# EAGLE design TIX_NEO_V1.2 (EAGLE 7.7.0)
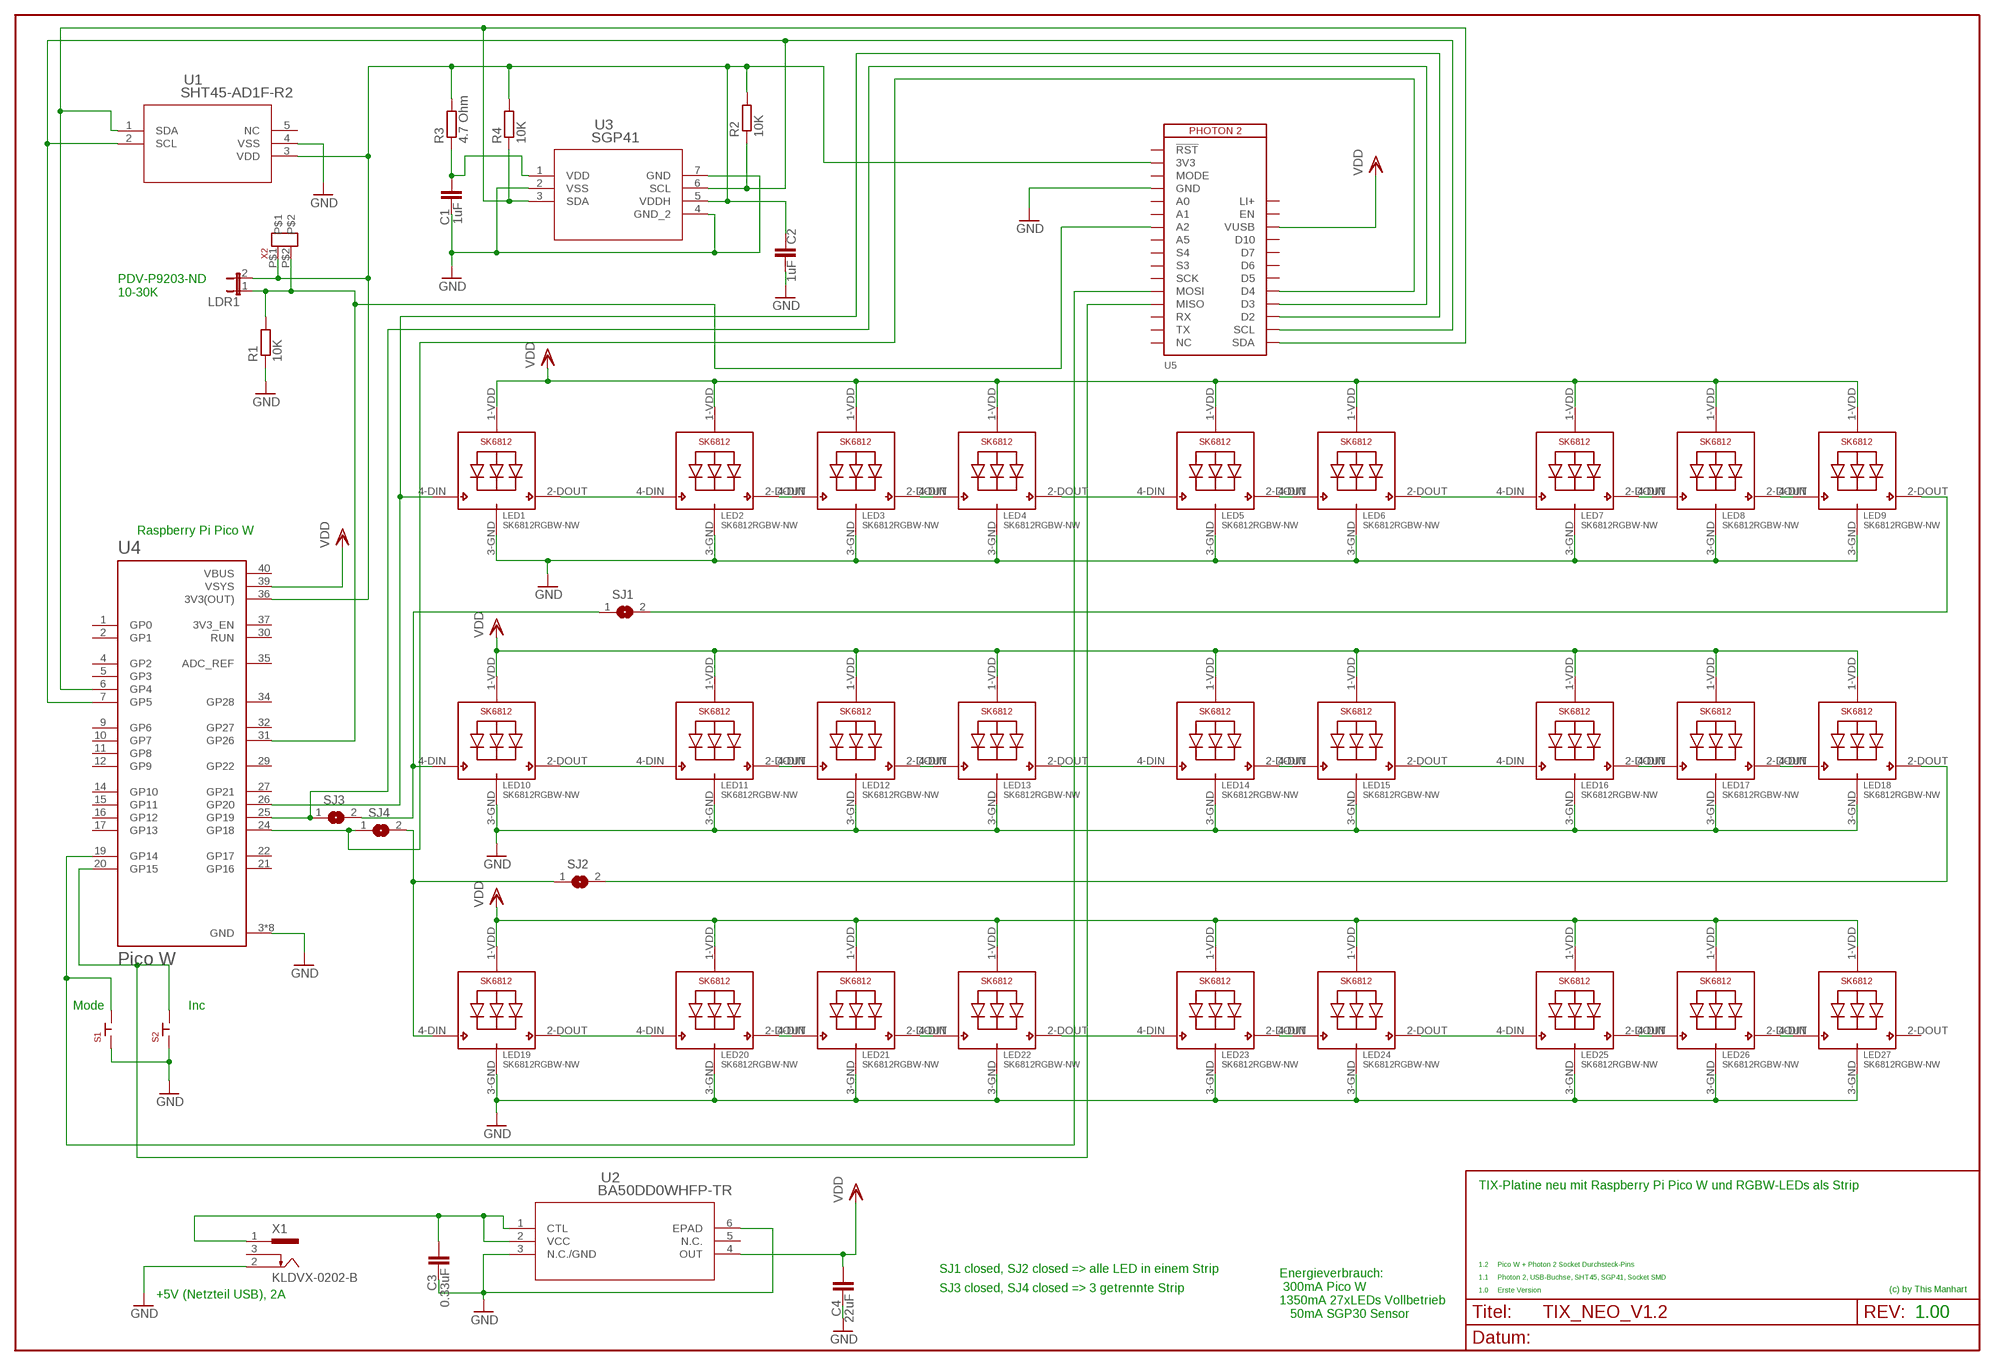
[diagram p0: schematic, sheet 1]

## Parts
C1  1uF  C-EUC0805  [C0805]
C2  1uF  C-EUC0805  [C0805]
C3  0.33uF  C-EUC0805  [C0805]
C4  22uF  C-EUC0805  [C0805]
LDR1  JUMPER_2P  [JUMPER_2P_2.54]
LED1  SK6812RGBW-NW  SK6812_5050W  [LED5050_W]
LED2  SK6812RGBW-NW  SK6812_5050W  [LED5050_W]
LED3  SK6812RGBW-NW  SK6812_5050W  [LED5050_W]
LED4  SK6812RGBW-NW  SK6812_5050W  [LED5050_W]
LED5  SK6812RGBW-NW  SK6812_5050W  [LED5050_W]
LED6  SK6812RGBW-NW  SK6812_5050W  [LED5050_W]
LED7  SK6812RGBW-NW  SK6812_5050W  [LED5050_W]
LED8  SK6812RGBW-NW  SK6812_5050W  [LED5050_W]
LED9  SK6812RGBW-NW  SK6812_5050W  [LED5050_W]
LED10  SK6812RGBW-NW  SK6812_5050W  [LED5050_W]
LED11  SK6812RGBW-NW  SK6812_5050W  [LED5050_W]
LED12  SK6812RGBW-NW  SK6812_5050W  [LED5050_W]
LED13  SK6812RGBW-NW  SK6812_5050W  [LED5050_W]
LED14  SK6812RGBW-NW  SK6812_5050W  [LED5050_W]
LED15  SK6812RGBW-NW  SK6812_5050W  [LED5050_W]
LED16  SK6812RGBW-NW  SK6812_5050W  [LED5050_W]
LED17  SK6812RGBW-NW  SK6812_5050W  [LED5050_W]
LED18  SK6812RGBW-NW  SK6812_5050W  [LED5050_W]
LED19  SK6812RGBW-NW  SK6812_5050W  [LED5050_W]
LED20  SK6812RGBW-NW  SK6812_5050W  [LED5050_W]
LED21  SK6812RGBW-NW  SK6812_5050W  [LED5050_W]
LED22  SK6812RGBW-NW  SK6812_5050W  [LED5050_W]
LED23  SK6812RGBW-NW  SK6812_5050W  [LED5050_W]
LED24  SK6812RGBW-NW  SK6812_5050W  [LED5050_W]
LED25  SK6812RGBW-NW  SK6812_5050W  [LED5050_W]
LED26  SK6812RGBW-NW  SK6812_5050W  [LED5050_W]
LED27  SK6812RGBW-NW  SK6812_5050W  [LED5050_W]
R1  10K  R-EU_R0805  [R0805]
R2  10K  R-EU_R0805  [R0805]
R3  4.7 Ohm  R-EU_R0805  [R0805]
R4  10K  R-EU_R0805  [R0805]
S1  TS02-66-170-BK-100-SCR-D  SCHURTER_LSH_PUSH_KEYDIP  [SCHURTER_LPH_PUSH_KEY]
S2  TS02-66-170-BK-100-SCR-D  SCHURTER_LSH_PUSH_KEYDIP  [SCHURTER_LPH_PUSH_KEY]
SJ1  SJ  [SJ]
SJ2  SJ  [SJ]
SJ3  SJ  [SJ]
SJ4  SJ  [SJ]
U1  SHT45-AD1F-R2  SHT40-AD1B-R2SHT4X_SEN-M  [SHT4X_SEN-M]
U2  BA50DD0WHFP-TR  BA50DD0WHFP-TRHRP5_ROM-M  [HRP5_ROM-M]
U3  SGP41  SGP41-D-R4DFN_SGP41-D-R4_SEN-M  [DFN_SGP41-D-R4_SEN-M]
U4  Pico W  RASPBERRY_PICO-NO_DEBUGW  [PICO-W]
U5  PHOTON2MM  [PHOTON2-MM]
X1  KLDVX-0202-B  [KLDVX-0202-B]
X2  PHOENIX_MPT_KLEMME_2P  [PHOENIX_MPT_KLEMME]

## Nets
GND: C1.1 C2.1 C3.1 C4.1 LED1.3-GND(GND) LED2.3-GND(GND) LED3.3-GND(GND) LED4.3-GND(GND) LED5.3-GND(GND) LED6.3-GND(GND) LED7.3-GND(GND) LED8.3-GND(GND) LED9.3-GND(GND) LED10.3-GND(GND) LED11.3-GND(GND) LED12.3-GND(GND) LED13.3-GND(GND) LED14.3-GND(GND) LED15.3-GND(GND) LED16.3-GND(GND) LED17.3-GND(GND) LED18.3-GND(GND) LED19.3-GND(GND) LED20.3-GND(GND) LED21.3-GND(GND) LED22.3-GND(GND) LED23.3-GND(GND) LED24.3-GND(GND) LED25.3-GND(GND) LED26.3-GND(GND) LED27.3-GND(GND) R1.1 S1.P$1 S2.P$1 U1.4(VSS) U2.3(N.C./GND) U2.6(EPAD) U3.2(VSS) U3.4(GND_2) U3.7(GND) U4.3(GND) U4.8(GND) U4.13(GND) U4.18(GND) U4.23(GND) U4.28(GND) U4.33(GND) U4.38(GND) U5.4(GND) X1.2
N$1: LED1.2-DOUT(DO) LED2.4-DIN(DI)
N$2: LED20.2-DOUT(DO) LED21.4-DIN(DI)
N$3: LED1.4-DIN(DI) U4.26(GP20) U5.19(D2)
N$4: LED2.2-DOUT(DO) LED3.4-DIN(DI)
N$5: LED3.2-DOUT(DO) LED4.4-DIN(DI)
N$6: LED4.2-DOUT(DO) LED5.4-DIN(DI)
N$7: LED5.2-DOUT(DO) LED6.4-DIN(DI)
N$8: LED6.2-DOUT(DO) LED7.4-DIN(DI)
N$9: LED7.2-DOUT(DO) LED8.4-DIN(DI)
N$10: LED8.2-DOUT(DO) LED9.4-DIN(DI)
N$11: LED9.2-DOUT(DO) SJ1.2
N$12: LED10.2-DOUT(DO) LED11.4-DIN(DI)
N$13: LED21.2-DOUT(DO) LED22.4-DIN(DI)
N$14: LED22.2-DOUT(DO) LED23.4-DIN(DI)
N$15: LED11.2-DOUT(DO) LED12.4-DIN(DI)
N$16: LED12.2-DOUT(DO) LED13.4-DIN(DI)
N$17: LED13.2-DOUT(DO) LED14.4-DIN(DI)
N$18: LED14.2-DOUT(DO) LED15.4-DIN(DI)
N$19: LED15.2-DOUT(DO) LED16.4-DIN(DI)
N$20: LED16.2-DOUT(DO) LED17.4-DIN(DI)
N$21: LED17.2-DOUT(DO) LED18.4-DIN(DI)
N$22: LED18.2-DOUT(DO) SJ2.2
N$23: LED23.2-DOUT(DO) LED24.4-DIN(DI)
N$24: LED24.2-DOUT(DO) LED25.4-DIN(DI)
N$25: LED19.2-DOUT(DO) LED20.4-DIN(DI)
N$26: LED25.2-DOUT(DO) LED26.4-DIN(DI)
N$27: LED26.2-DOUT(DO) LED27.4-DIN(DI)
N$28: LDR1.1 R1.2 U4.31(GP26) U5.7(A2) X2.P$2
N$29: C2.2 LDR1.2 R2.2 R3.2 R4.2 U1.3(VDD) U3.5(VDDH) U4.36(3V3(OUT)) U5.2(3V3) X2.P$1
N$31: S1.P$3 U4.19(GP14) U5.12(MOSI)
N$32: S2.P$3 U4.20(GP15) U5.13(MISO)
N$34: C1.2 R3.1 U3.1(VDD)
N$35: SJ4.1 U4.24(GP18) U5.21(D4)
N$36: LED19.4-DIN(DI) SJ2.1 SJ4.2
N$38: R2.1 U1.2(SCL) U3.6(SCL) U4.7(GP5) U5.18(SCL)
N$40: C3.2 U2.1(CTL) U2.2(VCC) X1.1
N$41: SJ3.1 U4.25(GP19) U5.20(D3)
N$42: LED10.4-DIN(DI) SJ1.1 SJ3.2
N$43: R4.1 U1.1(SDA) U3.3(SDA) U4.6(GP4) U5.17(SDA)
VDD: C4.2 LED1.1-VDD(VDD) LED2.1-VDD(VDD) LED3.1-VDD(VDD) LED4.1-VDD(VDD) LED5.1-VDD(VDD) LED6.1-VDD(VDD) LED7.1-VDD(VDD) LED8.1-VDD(VDD) LED9.1-VDD(VDD) LED10.1-VDD(VDD) LED11.1-VDD(VDD) LED12.1-VDD(VDD) LED13.1-VDD(VDD) LED14.1-VDD(VDD) LED15.1-VDD(VDD) LED16.1-VDD(VDD) LED17.1-VDD(VDD) LED18.1-VDD(VDD) LED19.1-VDD(VDD) LED20.1-VDD(VDD) LED21.1-VDD(VDD) LED22.1-VDD(VDD) LED23.1-VDD(VDD) LED24.1-VDD(VDD) LED25.1-VDD(VDD) LED26.1-VDD(VDD) LED27.1-VDD(VDD) U2.4(OUT) U4.39(VSYS) U5.26(VUSB)
Unconnected: LED27.2-DOUT(DO) U1.5(NC) U2.5(N.C.) U4.1(GP0) U4.2(GP1) U4.4(GP2) U4.5(GP3) U4.9(GP6) U4.10(GP7) U4.11(GP8) U4.12(GP9) U4.14(GP10) U4.15(GP11) U4.16(GP12) U4.17(GP13) U4.21(GP16) U4.22(GP17) U4.27(GP21) U4.29(GP22) U4.30(RUN) U4.32(GP27) U4.34(GP28) U4.35(ADC_REF) U4.37(3V3_EN) U5.1(!RST) U5.3(MODE) U5.5(A0) U5.6(A1) U5.8(A5) U5.9(S4) U5.10(S3) U5.11(SCK) U5.14(RX) U5.15(TX) U5.16(NC) U5.22(D5) U5.23(D6) U5.24(D7) U5.25(D10) U5.27(EN) X1.1@1 X1.2@1 X1.3 X1.3@1

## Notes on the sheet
- PDV-P9203-ND
  10-30K
- Raspberry Pi Pico W
- Mode | Inc
- TIX-Platine neu mit Raspberry Pi Pico W und RGBW-LEDs als Strip
- 1.2 | Pico W + Photon 2 Socket Durchsteck-Pins
- SJ1 closed, SJ2 closed => alle LED in einem Strip
- 1.1 | Photon 2, USB-Buchse, SHT45, SGP41, Socket SMD
- SJ3 closed, SJ4 closed => 3 getrennte Strip | 1.0 | Erste Version | (c) by This Manhart
- +5V (Netzteil USB), 2A
- Energieverbrauch:
   300mA Pico W
  1350mA 27xLEDs Vollbetrieb
     50mA SGP30 Sensor
- 1.00

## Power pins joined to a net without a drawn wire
LI+: U5.28(LI+)
VBUS: U4.40(VBUS)

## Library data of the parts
C1-C4 = rcl:C-EU: CAPACITOR, European symbol
LDR1 = 0_mm:JUMPER_2P
LED1-LED27 = SK6812:SK6812
R1-R4 = resistor:R-EU_: RESISTOR, European symbol
S1 S2 = 0_mm:SCHURTER_LSH_PUSH_KEY: Schurter 1301.932 - SMD Taster Farnell 309-5915
SJ1-SJ4 = jumper:SJ: SMD solder JUMPER
U1 = 0_mm:SHT40-AD1B-R2; COPYRIGHT: Copyright (C) 2024 Ultra Librarian. All rights reserved.; MANUFACTURER_PART_NUMBER: SHT40-AD1B-R2; MFR_NAME: Sensirion
U2 = rohm_semi:BA50DD0WHFP-TR; COPYRIGHT: Copyright (C) 2024 Ultra Librarian. All rights reserved.; MANUFACTURER_PART_NUMBER: BA50DD0WHFP-TR; MFR_NAME: ROHM Semiconductor
U3 = 0_mm:SGP41-D-R4; COPYRIGHT: Copyright (C) 2024 Ultra Librarian. All rights reserved.; MANUFACTURER_PART_NUMBER: SGP41-D-R4; MFR_NAME: Sensirion
U4 = RpiPico:RASPBERRY_PICO-NO_DEBUG
U5 = Particle-Devices:PHOTON2: Particle Photon 2 Wi-Fi enabled development kit Footprint and formfactor based on Adafruit Feather.
X1 = con-kycon_github:KLDVX-0202-: Power Jack, Vertical, PCB Mount, 2.0 mm, 2.5 mm, 3.0 mm Center Pin Source: KLDVX-0202x.pdf; OC_FARNELL: unknown; OC_NEWARK: unknown
X2 = 0_mm:PHOENIX_MPT_KLEMME_2P: Micro-Printklemme Raster 2.54mm

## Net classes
1 power: width 0.2 mm

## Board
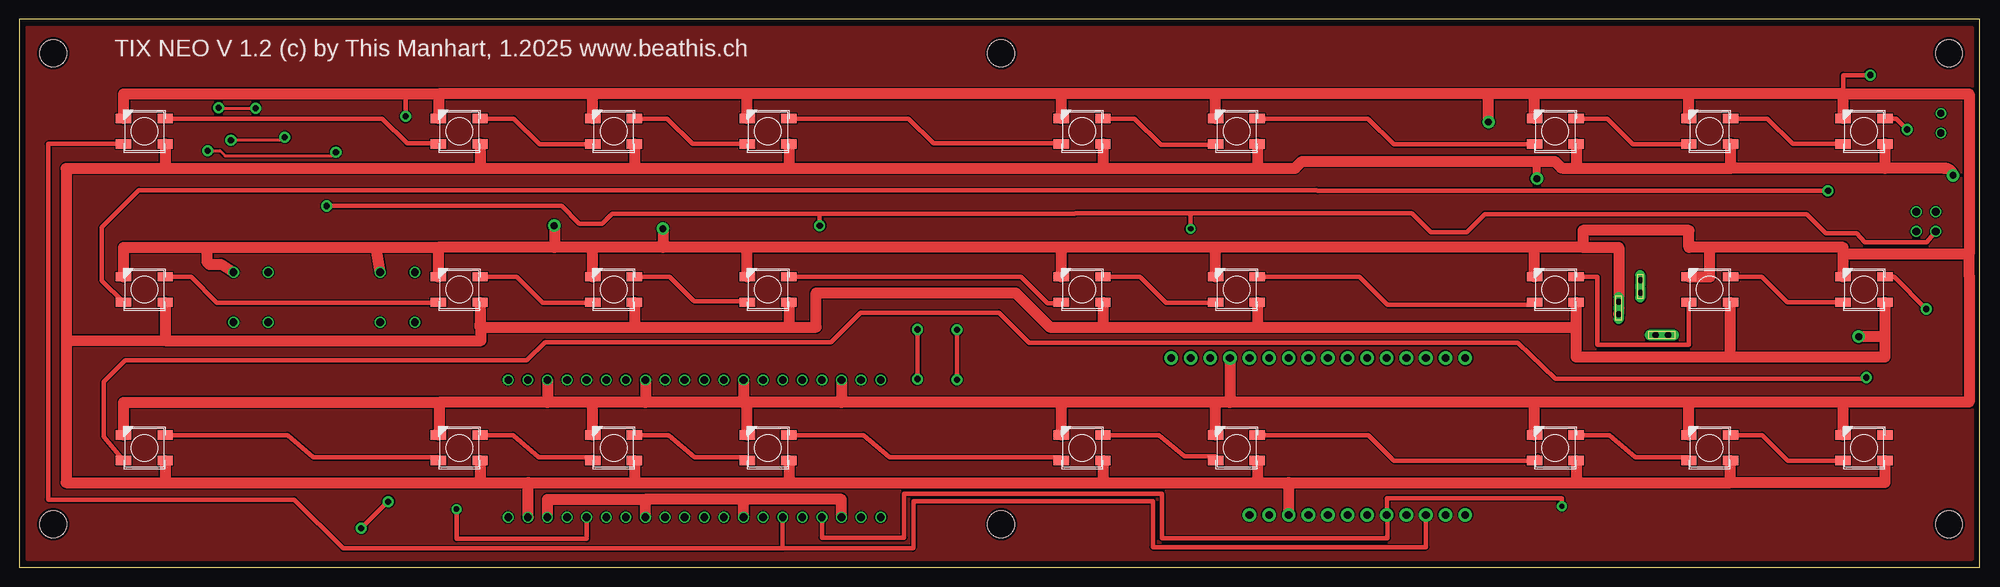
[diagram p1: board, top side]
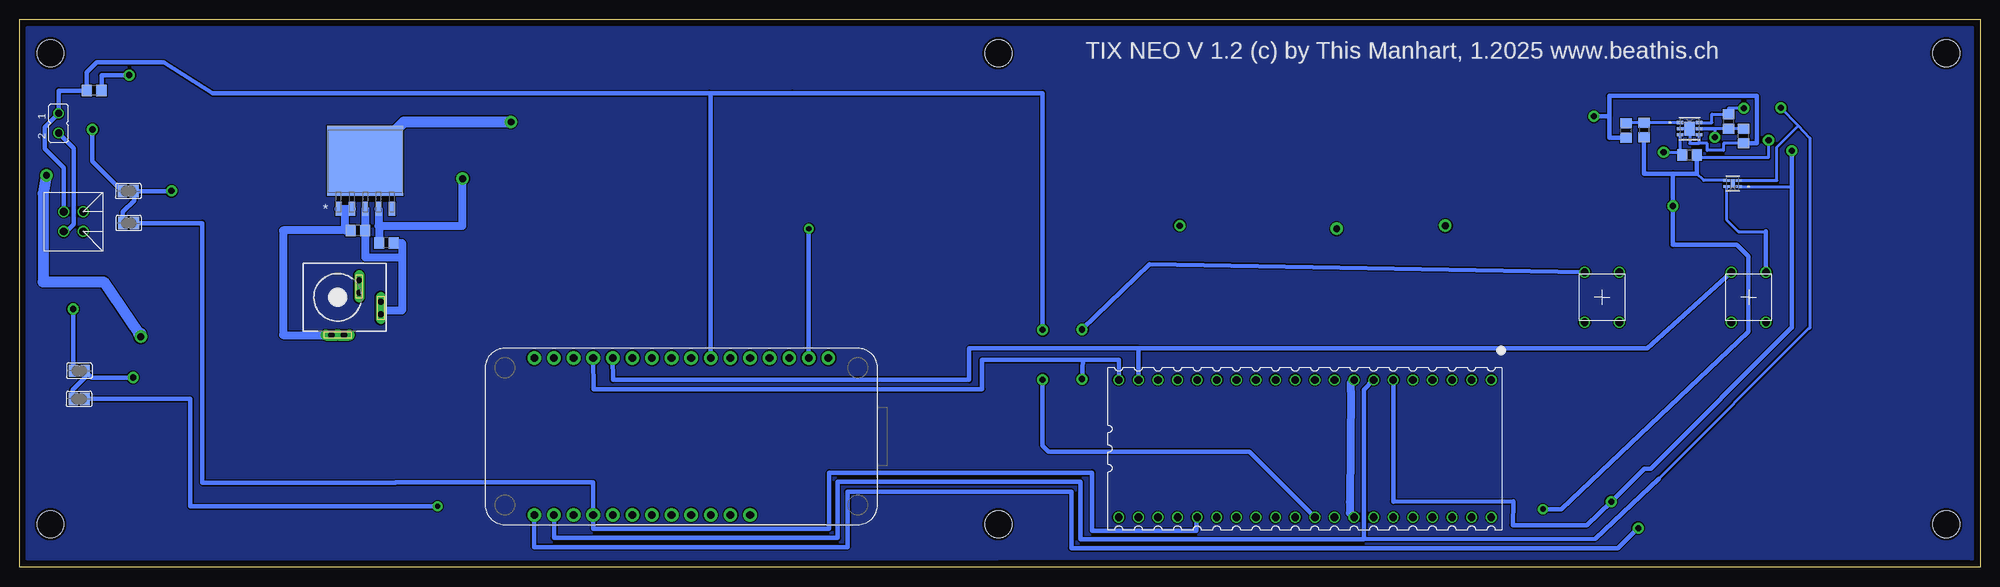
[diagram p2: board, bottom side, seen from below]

Size 254 x 71 mm. Coordinates in mm from the lower left corner, seen from the top.
Outline: 0,0 254,0 254,71 0,71 0,0
Copper layers (1*16): Top 0.035mm / dielectric 1.5mm / Bottom 0.035mm
Design rules "PCB-POOL Standard": minimum track width 0.15mm, minimum drill 0.3mm, track to track 0.15mm, track to pad 0.15mm, pad to pad 0.15mm, via to via 0.15mm, smd to smd 0.15mm, copper to edge 0.3mm, drill to drill 0.2mm, minimum pad ring 0.2mm, minimum via ring 0.15mm, stop-mask expansion 0.075mm, vias tented up to drill 0mil, thermal gap 0.2mm
Holes 3.5 mm at 4.4,5.6 4.4,66.6 127.2,5.6 127.2,66.6 250,5.6 250,66.6

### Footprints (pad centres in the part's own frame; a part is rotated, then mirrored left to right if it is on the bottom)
C0805 = smd 1.3 x 1.5: 1 -0.95,0; 2 0.95,0
JUMPER_2P_2.54 = drill 0.914: 1 -2.54,0; 2 0,0
LED5050_W = smd 2 x 1.2: 1-VDD 2.7,-1.65; 2-DOUT 2.7,1.65; 3-GND -2.7,1.65; 4-DIN -2.7,-1.65
R0805 = smd 1.3 x 1.5: 1 -0.95,0; 2 0.95,0
SCHURTER_LPH_PUSH_KEY = drill 1.016: P$1 -3.25,2.25; P$2 3.25,2.25; P$3 -3.25,-2.25; P$4 3.25,-2.25
SJ = smd 1.168 x 1.6: 1 -0.762,0; 2 0.762,0
SHT4X_SEN-M = smd 0.813 x 0.305: 1 -0.8,0.4; 2 -0.8,-0.4; 3 0.8,-0.4; 4 0.8,0.4 | smd 0.508 x 1.092: 5 0,0
HRP5_ROM-M = smd 0.787 x 1.854: 1 -3.454,-6.172; 2 -1.727,-6.172; 3 0,-6.172; 4 1.727,-6.172; 5 3.454,-6.172 | smd 9.855 x 9.017: 6 0,0.051
DFN_SGP41-D-R4_SEN-M = smd 0.864 x 0.406: 1 -1.245,0.8; 2 -1.245,0; 3 -1.245,-0.8; 4 1.245,-0.8; 5 1.245,0; 6 1.245,0.8 | smd 1.346 x 1.753: 7 0,0
PICO-W = drill 1: 1 -8.89,24.13; 2 -8.89,21.59; 3 -8.89,19.05; 4 -8.89,16.51; 5 -8.89,13.97; 6 -8.89,11.43; 7 -8.89,8.89; 8 -8.89,6.35; 9 -8.89,3.81; 10 -8.89,1.27; 11 -8.89,-1.27; 12 -8.89,-3.81; 13 -8.89,-6.35; 14 -8.89,-8.89; 15 -8.89,-11.43; 16 -8.89,-13.97; 17 -8.89,-16.51; 18 -8.89,-19.05; 19 -8.89,-21.59; 20 -8.89,-24.13; 21 8.89,-24.13; 22 8.89,-21.59; 23 8.89,-19.05; 24 8.89,-16.51; 25 8.89,-13.97; 26 8.89,-11.43; 27 8.89,-8.89; 28 8.89,-6.35; 29 8.89,-3.81; 30 8.89,-1.27; 31 8.89,1.27; 32 8.89,3.81; 33 8.89,6.35; 34 8.89,8.89; 35 8.89,11.43; 36 8.89,13.97; 37 8.89,16.51; 38 8.89,19.05; 39 8.89,21.59; 40 8.89,24.13
PHOTON2-MM = drill 1 pad 1.778: 1 1.27,44.45; 2 1.27,41.91; 3 1.27,39.37; 4 1.27,36.83; 5 1.27,34.29; 6 1.27,31.75; 7 1.27,29.21; 8 1.27,26.67; 9 1.27,24.13; 10 1.27,21.59; 11 1.27,19.05; 12 1.27,16.51; 13 1.27,13.97; 14 1.27,11.43; 15 1.27,8.89; 16 1.27,6.35; 17 21.59,6.35; 18 21.59,8.89; 19 21.59,11.43; 20 21.59,13.97; 21 21.59,16.51; 22 21.59,19.05; 23 21.59,21.59; 24 21.59,24.13; 25 21.59,26.67; 26 21.59,29.21; 27 21.59,31.75; 28 21.59,34.29
KLDVX-0202-B = drill 0.8 pad 1.4 long: 1 -4.9,0.8; 1@1 -4.9,-0.8 | drill 0.8 pad 1.3 long: 2 -2.2,-5.6; 2@1 -0.6,-5.6; 3 0.6,-2.8; 3@1 2.2,-2.8
PHOENIX_MPT_KLEMME = drill 1.016: P$1 2.54,0; P$2 2.54,-2.54; P$3 0,-2.54; P$4 0,0

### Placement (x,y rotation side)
C1  45.88,56.6 90 bottom
C2  30.65,55.88 90 bottom
C3  210.18,43.65 180 bottom
C4  206.47,42.05 180 bottom
LDR1  248.97,56.27 270 bottom
LED1  16.2,56.5 0 top
LED2  57,56.5 0 top
LED3  77,56.5 0 top
LED4  97,56.5 0 top
LED5  137.7,56.5 0 top
LED6  157.7,56.5 0 top
LED7  199,56.5 0 top
LED8  219,56.5 0 top
LED9  239,56.5 0 top
LED10  16.2,36 0 top
LED11  57,36 0 top
LED12  77,36 0 top
LED13  97,36 0 top
LED14  137.7,36 0 top
LED15  157.7,36 0 top
LED16  199,36 0 top
LED17  219,36 0 top
LED18  239,36 0 top
LED19  16.2,15.5 0 top
LED20  57,15.5 0 top
LED21  77,15.5 0 top
LED22  97,15.5 0 top
LED23  137.7,15.5 0 top
LED24  157.7,15.5 0 top
LED25  199,15.5 0 top
LED26  219,15.5 0 top
LED27  239,15.5 0 top
R1  244.35,61.77 180 bottom
R2  32.62,57.77 270 bottom
R3  43.55,56.65 270 bottom
R4  37.65,53.45 0 bottom
S1  30,35 270 bottom
S2  49,35 270 bottom
SJ1  239.93,48.75 180 bottom
SJ2  246.28,25.48 180 bottom
SJ3  239.88,44.6 180 bottom
SJ4  246.3,21.82 180 bottom
U1  32.08,49.73 180 bottom
U2  209.22,52.62 0 bottom
U3  37.65,56.83 0 bottom
U4  87.47,15.4 270 bottom
U5  193.68,28.4 270 bottom
X1  212.8,35 90 bottom
X2  245.75,43.52 180 bottom

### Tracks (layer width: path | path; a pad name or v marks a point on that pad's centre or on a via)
GND  (via drill 0.8 pad 1.02, 0.8 pad 1.27, 0.9 pad 1.27)
  Top 0.61: 236.3,61.35 236.3,63.77 v239.8,63.77 | v50.05,58.42 50.05,61.35 49.85,61.35
  Top 1.422: LED1.3-GND 13.5,61.35 49.85,61.35 54.3,61.35 | 54.3,61.35 LED2.3-GND | LED3.3-GND 74.3,61.35 | 74.3,61.35 54.3,61.35 | LED4.3-GND 94.3,61.35 | 94.3,61.35 74.3,61.35 | LED5.3-GND 135,61.35 | 135,61.35 94.3,61.35 | LED6.3-GND 155,61.35 | 155,61.35 135,61.35 | LED7.3-GND 196.3,61.35 | 196.3,61.35 190.35,61.35 | 190.35,61.35 155,61.35 | LED8.3-GND 216.3,61.35 | 216.3,61.35 196.3,61.35 | LED9.3-GND 236.3,61.35 | 236.3,61.35 216.3,61.35 | LED10.3-GND 13.5,41.48 24.32,41.48 | 24.32,41.48 46.17,41.48 | 46.17,41.48 54.25,41.48 | 54.25,41.48 54.25,37.65 LED11.3-GND | LED12.3-GND 74.3,41.48 | 74.3,41.48 69.33,41.48 | 69.33,41.48 54.25,41.48 | LED13.3-GND 94.3,41.48 | 94.3,41.48 83.38,41.48 | 83.38,41.48 74.3,41.48 | LED14.3-GND 135,41.48 | 135,41.48 94.3,41.48 | LED15.3-GND 155,41.48 | 155,41.48 135,41.48 | LED16.3-GND 196.3,41.48 | 196.3,41.48 155,41.48 | 202.6,41.48 202.6,43.65 216.3,43.65 216.3,41.48 219.05,41.48 | 202.6,41.48 196.3,41.48 | LED18.3-GND 236.3,40.55 | 236.3,40.55 236.3,41.48 219.05,41.48 | LED19.3-GND 13.5,21.38 54.38,21.38 | 54.38,21.38 54.38,17.65 LED20.3-GND | LED21.3-GND 74.3,21.38 | 74.3,21.38 68.42,21.38 | 68.42,21.38 54.38,21.38 | LED22.3-GND 94.3,21.38 | 94.3,21.38 93.83,21.38 | 93.83,21.38 81.12,21.38 | 81.12,21.38 74.3,21.38 | LED23.3-GND 135,21.38 | 135,21.38 106.53,21.38 | 106.53,21.38 94.3,21.38 | LED24.3-GND 155,21.38 | 155,21.38 135,21.38 | LED25.3-GND 196.3,21.38 | 196.3,21.38 156.84,21.38 | 156.84,21.38 155,21.38 | LED26.3-GND 216.3,21.38 | 216.3,21.38 196.3,21.38 | LED27.3-GND 236.3,21.38 | 236.3,21.38 216.3,21.38 | 236.3,61.35 252.6,61.35 252.6,40.55 | 252.6,40.55 236.3,40.55 | 236.3,21.38 252.62,21.43 252.62,37.85 252.6,37.8 252.6,40.55
  Top 1.422: S1.P$1 26.12,39.25 26.1,39.23 24.65,39.23 24.32,39.55 24.32,41.48 | v83.38,43.88 83.38,41.48 | v69.3,44.27 69.33,44.27 69.33,41.48 | LED17.3-GND 219.05,37.65 219.05,41.48 | S2.P$1 46.25,41.4 46.17,41.48 | 202.6,41.48 207.2,41.48 X1.2 | v190.35,57.7 190.35,61.35 | U4.3 68.42,21.38 | U4.8 81.12,21.38 | U4.13 93.83,21.38 | U4.18 106.53,21.38 | U4.38 68.42,8.82 81.1,8.82 | 81.1,8.82 81.1,6.51 U4.33 | U4.28 93.83,8.82 | 93.83,8.82 81.1,8.82 | U4.23 106.53,8.82 93.83,8.82 | U5.4 156.84,21.38
  Bottom 0.406: C2.1 33.25,54.92 33.25,54.02 35.38,54.02 35.38,54.92 36.41,54.92 | 36.41,54.92 U3.4 | 36.41,54.92 37.65,54.92 U3.7 U3.2 | U1.4 32.88,45.05 31.32,43.5 27.77,43.5 27.75,43.52
  Bottom 0.61: v239.8,63.77 243.4,63.77 R1.1 | 27.75,43.52 S1.P$1 | C1.1 48.05,55.65 48.05,58.42 | C2.1 30.65,54.95 28.95,54.95 28.95,61.08 48.05,61.08 48.05,58.42 | 48.05,58.42 v50.05,58.42
  Bottom 1.016: U2.3 C3.1 209.22,40.17 204.47,40.17 | C4.1 204.47,42.05 204.47,40.17 | 204.47,40.17 204.47,33.27 207.2,33.27 X1.2 | U4.8 81.55,23.86 81.55,22.88 81.67,8.45 81.67,7.06 U4.33
  Bottom 1.422: 83.4,43.88 v83.38,43.88 | 209.2,52.68 U2.6 204.2,57.7 v190.35,57.7
N$1
  Top 0.61: LED1.2-DOUT 47,58.15 50.23,54.92 54.23,54.92 LED2.4-DIN
N$2
  Top 0.61: LED20.2-DOUT 63.95,17.15 67.3,14.3 74.25,14.3 LED21.4-DIN
N$3
  Top 0.61: LED1.4-DIN 3.73,54.85 3.73,8.8 35.62,8.8 41.95,2.48 98.91,2.48 | 98.91,2.48 U4.26 | 98.91,2.48 115.72,2.48 115.83,2.58 115.83,8.57 146.85,8.57 146.85,2.65 182.25,2.65 U5.19
N$4
  Top 0.61: LED2.2-DOUT 64.08,58.15 67.42,54.8 74.25,54.8 LED3.4-DIN
N$5
  Top 0.61: LED3.2-DOUT 83.95,58.15 87.25,54.85 LED4.4-DIN
N$6
  Top 0.61: LED4.2-DOUT 115.2,58.15 118.42,54.92 134.93,54.92 LED5.4-DIN
N$7
  Top 0.61: LED5.2-DOUT 144.5,58.15 147.93,54.73 154.88,54.73 LED6.4-DIN
N$8
  Top 0.61: LED6.2-DOUT 174.75,58.15 178.07,54.83 196.28,54.83 LED7.4-DIN
N$9
  Top 0.61: LED7.2-DOUT 205.72,58.15 209.07,54.8 216.25,54.8 LED8.4-DIN
N$10
  Top 0.61: LED8.2-DOUT 226.47,58.15 229.78,54.85 LED9.4-DIN
N$11  (via drill 0.8 pad 1.27)
  Top 0.61: LED9.2-DOUT 243.15,58.15 v244.57,56.73
  Bottom 0.61: v244.57,56.73 244.57,52.64 SJ1.2
N$12
  Top 0.61: LED10.2-DOUT 22.25,37.62 25.6,34.27 54.25,34.3 LED11.4-DIN
N$13
  Top 0.61: LED21.2-DOUT 84.1,17.15 87.5,14.25 94.3,14.25 | 94.4,14.25 94.3,14.25 | 94.3,14.25 LED22.4-DIN
N$14
  Top 0.61: LED22.2-DOUT 109.38,17.15 112.78,14.28 134.9,14.25 LED23.4-DIN
N$15
  Top 0.61: LED11.2-DOUT 64.45,37.65 67.8,34.3 74.25,34.3 LED12.4-DIN
N$16
  Top 0.61: LED12.2-DOUT 84.28,37.65 87.42,34.5 94.15,34.5 LED13.4-DIN
N$17
  Top 0.61: LED13.2-DOUT 129.78,37.65 133.2,34.23 134.88,34.23 LED14.4-DIN
N$18
  Top 0.61: LED14.2-DOUT 145.18,37.65 148.53,34.3 154.95,34.3 LED15.4-DIN
N$19
  Top 0.61: LED15.2-DOUT 173.65,37.65 177.25,34.05 196,34.05 LED16.4-DIN
N$20
  Top 0.61: LED16.2-DOUT 204.47,37.65 204.47,28.82 216.3,28.82 LED17.4-DIN
N$21
  Top 0.61: LED17.2-DOUT 225.78,37.65 229.07,34.35 LED18.4-DIN
N$22  (via drill 0.8 pad 1.27)
  Top 0.61: LED18.2-DOUT 242.9,37.65 v247.07,33.48
  Bottom 0.61: v247.07,33.48 247.07,25.51 SJ2.2
N$23
  Top 0.61: LED23.2-DOUT 147.65,17.15 150.93,14.38 154.97,14.38 LED24.4-DIN
N$24
  Top 0.61: LED24.2-DOUT 174.78,17.15 178.07,13.85 LED25.4-DIN | LED25.4-DIN 196.75,14.35 196.88,14.22 196.43,14.22 LED25.4-DIN
N$25
  Top 0.61: LED19.2-DOUT 34.75,17.15 38.1,14.3 54.25,14.3 LED20.4-DIN
N$26
  Top 0.61: LED25.2-DOUT 206.03,17.15 209.4,14.28 216.22,14.28 LED26.4-DIN
N$27
  Top 0.61: LED26.2-DOUT 225.8,17.15 229.1,13.85 LED27.4-DIN
N$28  (via drill 0.8 pad 1.02)
  Top 0.61: v121.47,24.32 v121.47,30.77
  Bottom 0.61: 164.62,61.44 228.97,61.4 235.35,65.42 244.03,65.42 245.3,64.15 R1.2 248.97,61.77 LDR1.1 250.75,57.02 250.75,54.25 248.29,51.79 X2.P$2 | 164.62,61.44 153.93,61.45 121.47,61.45 v121.47,30.77 | U4.31 94.69,15 120.7,15 121.47,15.78 v121.47,24.32 | U5.7 164.47,61.28 164.62,61.44
N$29  (via drill 0.7 pad 1.02, 0.8 pad 1.02, 0.8 pad 1.27)
  Top 0.406: v34.4,55.73 34.4,55.35 v27.43,55.35
  Top 0.61: 151.75,45.85 180.43,45.85 182.85,43.42 187.53,43.42 189.88,45.77 231.55,45.77 234.05,43.27 238.07,43.27 239.1,42.1 247.12,42.1 X2.P$1 | 151.75,45.85 136.82,45.85 136.78,45.8 103.7,45.8 | 103.7,45.8 76.78,45.8 75.53,44.55 72.55,44.55 70.25,46.85 39.85,46.85 v39.83,46.83 | v103.7,44.27 103.7,45.8 | U4.36 73.5,3.7 56.65,3.7 v56.65,7.55 | v151.75,43.88 151.75,45.85
  Bottom 0.406: C2.2 R2.2 U3.5 34.4,56.83 v34.4,55.73 | v27.43,55.35 27.43,53.08 36.7,53.08 R4.2 | U1.3 35.83,50.12 36.7,51
  Bottom 0.61: 103.72,44.26 v103.7,44.27 | R4.2 36.7,51 39.77,51 | R3.2 43.55,51 39.77,51 | X2.P$1 247.9,43.52 246.97,44.45 246.97,54.28 LDR1.2 | 39.77,51 39.83,50.95 v39.83,46.83 39.83,41.8 39.85,41.77 31.5,41.77 30.02,40.3 30.02,30.55 54.25,7.55 v56.65,7.55 | U5.2 151.76,43.86 v151.75,43.88
N$31
  Bottom 0.61: 109.06,28.38 U4.19 | 109.06,28.38 43.12,28.38 S1.P$3 | 109.06,28.38 131,28.38 130.97,24.3 177.14,24.3 U5.12
N$32  (via drill 0.8 pad 1.02)
  Top 0.61: v116.35,30.82 v116.35,24.4
  Bottom 0.61: 116.22,26.9 111.58,26.9 111.58,24.29 U4.20 | S2.P$3 107.6,39.25 v116.35,30.82 | v116.35,24.4 116.22,26.9 | U5.13 179.66,23.1 129.3,23.1 129.35,26.9 116.22,26.9
N$33
  pour Bottom: 1.45,1.15 253,1 253,70 1,70 1,1
N$34
  Bottom 0.406: U3.1 43.55,57.62 R3.1 45.88,57.6 C1.2
N$35  (via drill 0.7 pad 1.02)
  Top 0.61: U4.24 103.98,3.88 114.65,3.88 114.65,9.57 148.03,9.57 148.03,3.8 177.28,3.8 177.28,6.81 U5.21 177.15,6.81 177.15,8.95 199.85,8.95 v199.85,7.92
  Bottom 0.61: SJ4.1 231.9,21.82 231.9,7.92 v199.85,7.92
N$36  (via drill 0.8 pad 1.27)
  Top 0.61: LED19.4-DIN 10.95,16.9 10.95,24.07 13.7,26.82 65.75,26.82 68.1,29.18 105.17,29.18 109,33 126.9,33 130.82,29.07 194.18,29.1 199.03,24.45 239.15,24.45 v239.3,24.6
  Bottom 0.61: SJ4.2 247.12,21.89 247.12,23.05 245.51,24.66 SJ2.1 244.64,24.6 v239.3,24.6
N$37
  pour Top: 1,70 253,70 253,1 1,1
N$38  (via drill 0.8 pad 1.27)
  Top 0.406: v25.82,59.52 25.95,59.5 v30.62,59.5
  Bottom 0.406: 41.65,11.5 22.18,30.98 arc-90 22.07,31.07 22.07,55.62 23.59,57.2 | U3.6 34.75,57.62 34.75,58.73 R2.1 32.62,59.5 v30.62,59.5 | 23.59,57.2 v25.82,59.52 | U1.2 26.35,50.12 26.35,54.44 23.59,57.2
  Bottom 0.61: 79.88,3.62 116.55,3.62 116.55,11.07 148.03,11.07 148.03,3.83 184.78,3.83 U5.18 | 79.88,3.62 49.88,3.75 41.65,11.5 | U4.7 79.88,23 79.88,3.62
N$40
  Bottom 1.016: 210.95,43.65 C3.2 211.8,43.65 | U2.1 211.8,46.45 | 211.8,46.45 U2.2 | 211.8,43.65 211.8,46.45 | 211.8,43.65 219.88,43.65 219.88,30.1 X1.1
N$41
  Bottom 0.61: U4.25 101.55,6.51 101.55,4.78 115.05,4.78 115.08,12.28 149.12,12.28 149.12,5.03 179.71,5.03 U5.20 179.71,11.03 205.28,11.03 205.28,10.97 230.35,10.97 230.35,44.6 SJ3.1
N$42  (via drill 0.8 pad 1.27)
  Top 0.61: LED10.4-DIN 10.7,37.15 10.7,44.08 15.5,48.88 168.1,48.88 168.2,48.77 v234.32,48.77
  Bottom 0.61: SJ3.2 240.62,44.61 240.62,46.05 239.16,47.51 SJ1.1 234.35,48.75 v234.32,48.77
N$43  (via drill 0.8 pad 1.02, 0.8 pad 1.27)
  Top 0.406: v24.43,53.98 26,53.98 26.68,53.3 40.52,53.3 v41.02,53.8
  Top 0.61: v44.3,5.1 47.73,8.53 v47.8,8.53
  Bottom 0.406: 24.43,31.05 arc90 24.45,31.02 | U3.3 38.9,53.45 R4.1 38.95,53.8 v41.02,53.8 | U1.1 24.43,49.33
  Bottom 0.61: v24.43,53.98 24.43,49.33 24.43,31.05 | 24.45,31.02 42.67,12.8 43.52,12.8 v47.8,8.53 50.95,5.5 60.55,5.47 60.5,8.57 76.05,8.53 U4.6 | v44.3,5.1 44.33,5.1 46.92,2.5 117.75,2.5 117.75,9.82 146.75,9.82 146.75,2.65 187.32,2.65 U5.17
VDD  (via drill 0.9 pad 1.27, 0.9 pad 1.42)
  Top 1.016: v196.62,50.38 196.62,52.6
  Top 1.422: LED9.1-VDD 241.7,51.7 | 241.7,51.7 221.72,51.7 | 221.72,51.7 221.72,54.85 LED8.1-VDD | LED7.1-VDD 201.7,51.7 | 201.7,51.7 221.72,51.7 | LED6.1-VDD 160.4,51.7 | 160.4,51.7 165.28,51.7 166.18,52.6 196.62,52.6 198.93,52.6 199.78,51.75 200.1,51.7 201.7,51.7 | LED5.1-VDD 140.4,51.7 | 140.4,51.7 160.4,51.7 | LED4.1-VDD 99.7,51.7 | 99.7,51.7 140.4,51.7 | LED3.1-VDD 79.7,51.7 | 79.7,51.7 99.7,51.7 | LED2.1-VDD 59.7,51.7 | 59.7,51.7 79.7,51.7 | LED1.1-VDD 18.9,51.7 | 18.9,51.7 59.7,51.7 | 221.7,27.25 241.7,27.25 LED18.1-VDD 241.7,29.9 v238.3,29.9 | 221.7,27.25 LED17.1-VDD | 221.7,27.25 201.7,27.25 201.7,31.12 | 201.7,31.12 LED16.1-VDD | LED15.1-VDD 160.4,31.12 | 160.4,31.12 201.7,31.12 | LED14.1-VDD 140.4,31.12 | 140.4,31.12 160.4,31.12 | LED13.1-VDD 99.7,31.12 | 99.7,31.12 103.25,31.12 103.25,35.58 129.07,35.58 133.53,31.12 140.4,31.12 | LED12.1-VDD 79.7,31.12 | 79.7,31.12 99.7,31.12 | LED11.1-VDD 59.7,31.48 | 59.7,31.48 59.7,31.12 79.7,31.12 | LED10.1-VDD 18.9,29.38 | 18.9,29.38 59.83,29.38 59.83,31.48 59.7,31.48 | LED27.1-VDD 241.7,11 221.7,11 | 221.7,11 LED26.1-VDD | LED25.1-VDD 201.7,11 | 201.7,11 221.7,11 | LED24.1-VDD 160.4,11 | 160.4,11 164.47,11 | 164.47,11 201.7,11 | LED23.1-VDD 140.4,11 | 140.4,11 160.4,11 | LED22.1-VDD 99.7,11 | 99.7,11 140.4,11 | LED21.1-VDD 79.7,11 | 79.7,11 99.7,11 | LED20.1-VDD 59.7,11 | 59.7,11 65.92,11 | 65.92,11 79.7,11 | LED19.1-VDD 18.9,11 | 18.9,11 59.7,11 | 18.9,11 18.88,10.97 6.05,10.97 6.05,51.7 18.9,51.7 | 6.28,29.4 18.9,29.38 | v250.53,50.8 arc90 249.35,51.7 241.7,51.7 | U4.39 65.92,6.51 65.92,11 | U5.26 164.47,11
  Bottom 1.016: 207.5,42.05 C4.2 207.43,44.25 | U2.4 207.5,44.25 207.43,44.25 | 207.43,44.25 196.62,44.25 v196.62,50.38
  Bottom 1.422: v250.53,50.8 250.97,48.45 250.97,36.98 243.12,37 238.58,30.32 | 238.58,30.32 v238.3,29.9 238.3,30.32 238.58,30.32

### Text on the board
tNames: TIX NEO V 1.2 (c) by This Manhart, 1.2025 www.beathis.ch
bNames: TIX NEO V 1.2 (c) by This Manhart, 1.2025 www.beathis.ch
